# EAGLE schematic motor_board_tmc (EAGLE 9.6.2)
Assembly variants: ACS724, MAX503xD+ACS

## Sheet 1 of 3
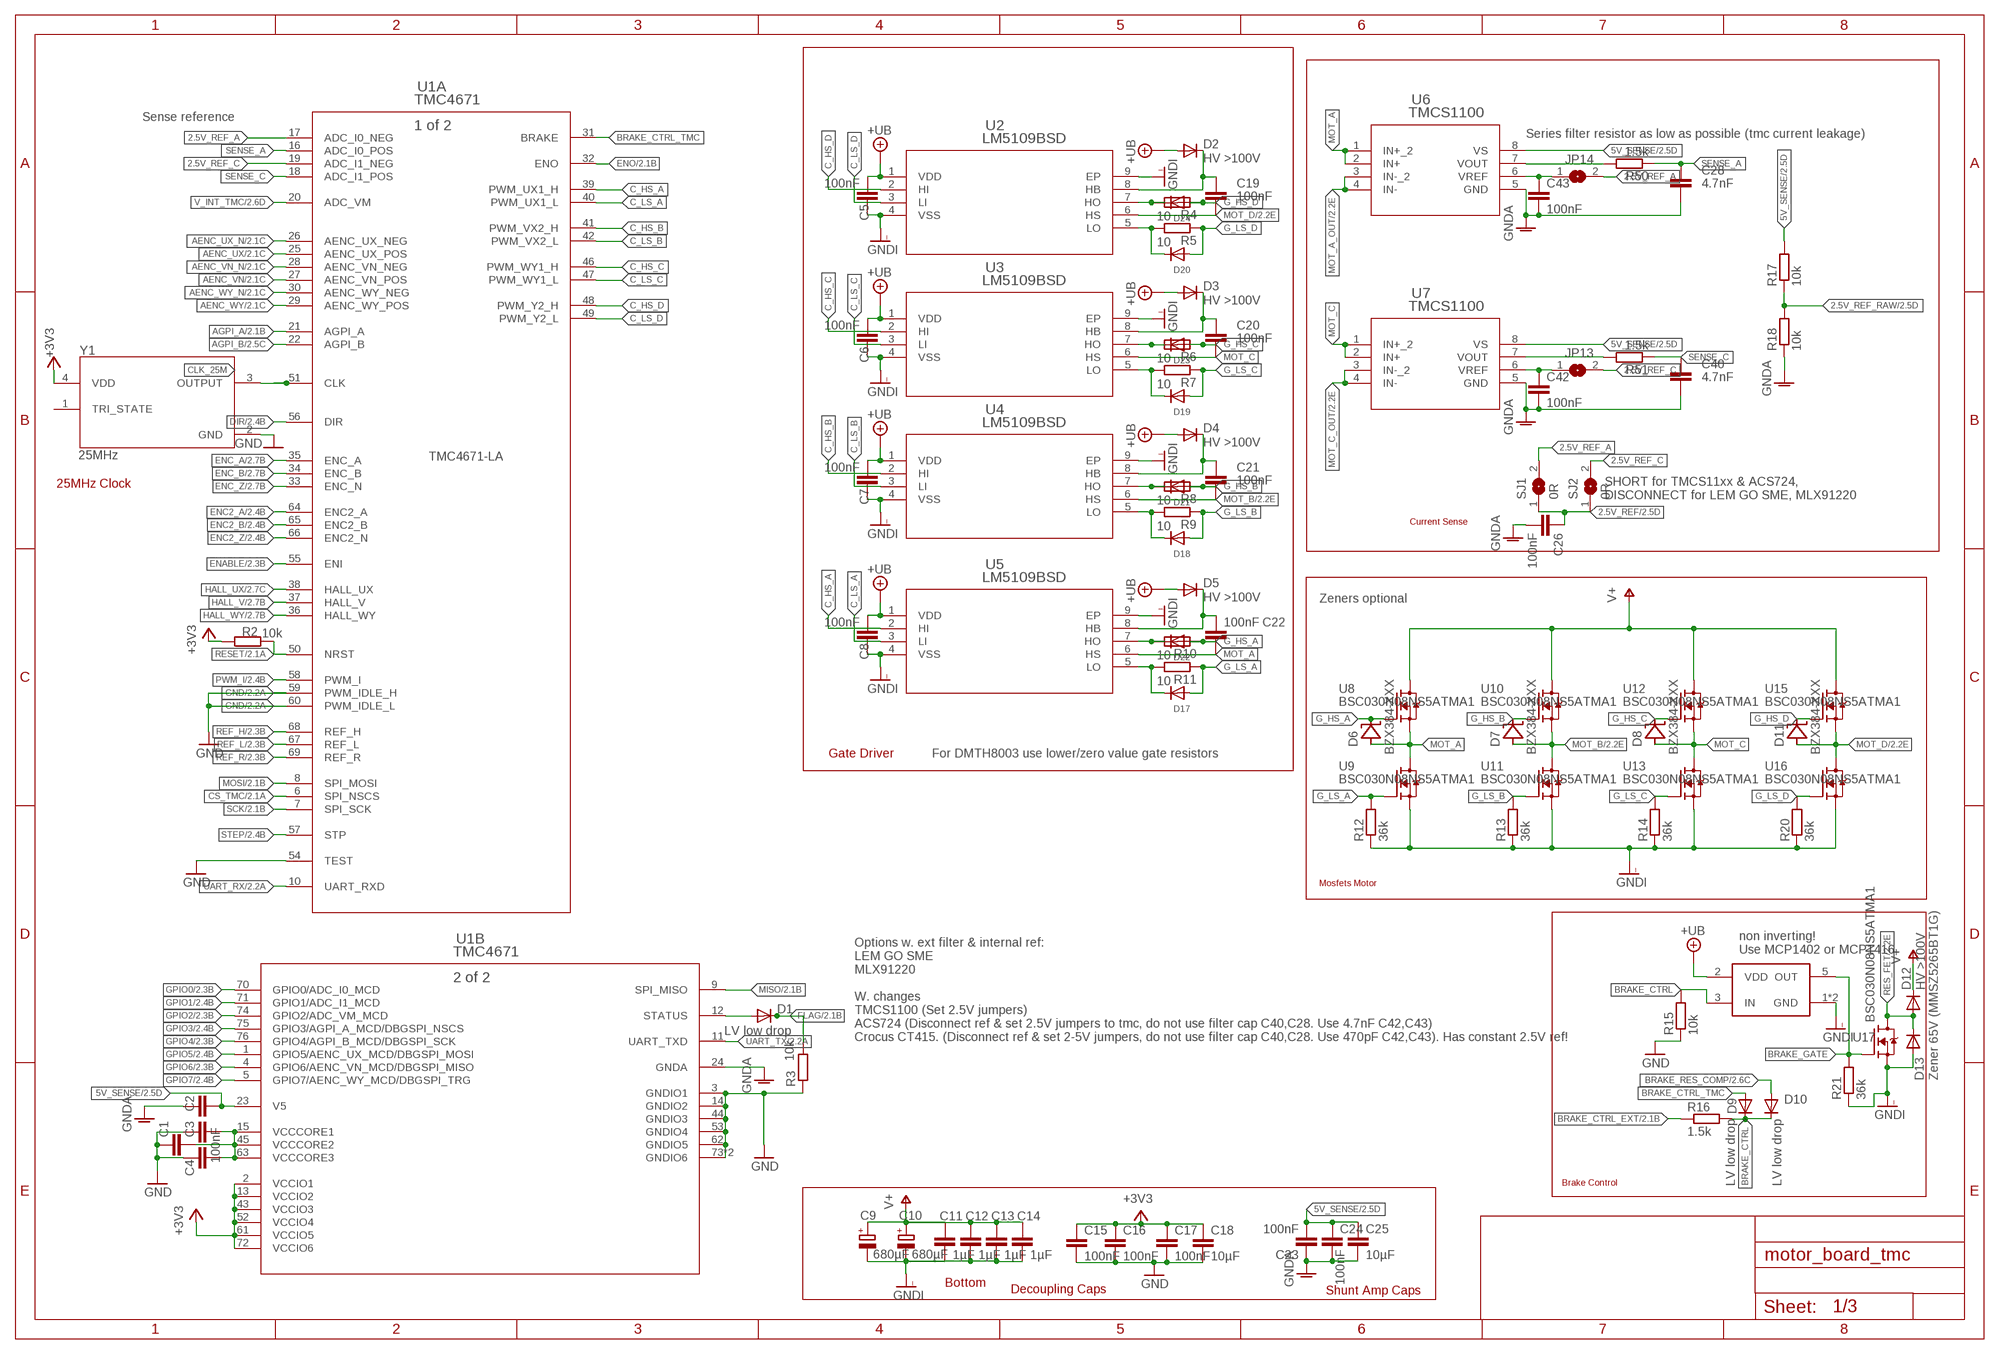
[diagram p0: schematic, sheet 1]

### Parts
C1  100nF  C-EUC0603  [C0603]
C2  10µF  C-EUC0805  [C0805]
C3  100nF  C-EUC0603  [C0603]
C4  100nF  C-EUC0603  [C0603]
C5  100nF  C-EUC0603  [C0603]
C6  100nF  C-EUC0603  [C0603]
C7  100nF  C-EUC0603  [C0603]
C8  100nF  C-EUC0603  [C0603]
C9  680µF  CPOL-EUE7.5-16  [E7,5-16]
C10  680µF  CPOL-EUE7.5-16  [E7,5-16]
C11  1µF  C-EUC1206  [C1206]
C12  1µF  C-EUC1206  [C1206]
C13  1µF  C-EUC1206  [C1206]
C14  1µF  C-EUC1206  [C1206]
C15  100nF  C-EUC0603  [C0603]
C16  100nF  C-EUC0603  [C0603]
C17  100nF  C-EUC0603  [C0603]
C18  10µF  C-EUC0805  [C0805]
C19  100nF  C-EUC0603  [C0603]
C20  100nF  C-EUC0603  [C0603]
C21  100nF  C-EUC0603  [C0603]
C22  100nF  C-EUC0603  [C0603]
C23  100nF  C-EUC0603  [C0603]
C24  100nF  C-EUC0603  [C0603]
C25  10µF  C-EUC0805  [C0805]
C26  100nF  C-EUC0603  [C0603]
C28  4.7nF  C-EUC0603  [C0603]  (not fitted in variant ACS724)  (not fitted in variant MAX503xD+ACS)
C40  4.7nF  C-EUC0603  [C0603]  (not fitted in variant ACS724)  (not fitted in variant MAX503xD+ACS)
C42  100nF  C-EUC0603  [C0603]  (variant ACS724: 4.7nF)  (variant MAX503xD+ACS: 4.7nF)
C43  100nF  C-EUC0603  [C0603]  (variant ACS724: 4.7nF)  (variant MAX503xD+ACS: 4.7nF)
D1  LV low drop  DIODE_SOD-123FL  [SOD-123FL]
D2  HV >100V  DIODE_SOD-123FL  [SOD-123FL]
D3  HV >100V  DIODE_SOD-123FL  [SOD-123FL]
D4  HV >100V  DIODE_SOD-123FL  [SOD-123FL]
D5  HV >100V  DIODE_SOD-123FL  [SOD-123FL]
D6  BZX384-XXX  [SOD323-R]
D7  BZX384-XXX  [SOD323-R]
D8  BZX384-XXX  [SOD323-R]
D9  LV low drop  DIODE_SOD-123FL  [SOD-123FL]
D10  LV low drop  DIODE_SOD-123FL  [SOD-123FL]
D11  BZX384-XXX  [SOD323-R]
D12  HV >100V  DIODE_SOD-123FL  [SOD-123FL]
D13  Zener 65V (MMSZ5265BT1G)  DIODE_SOD-123FL  [SOD-123FL]
D17  DIODESOD-323F  [SOD-323F]
D18  DIODESOD-323F  [SOD-323F]
D19  DIODESOD-323F  [SOD-323F]
D20  DIODESOD-323F  [SOD-323F]
D21  DIODESOD-323F  [SOD-323F]
D22  DIODESOD-323F  [SOD-323F]
D23  DIODESOD-323F  [SOD-323F]
D24  DIODESOD-323F  [SOD-323F]
JP13  JUMPER-SMT_2_NO_SILK  RESJUMPER0603  [RESISTOR_R0603]  (not fitted in variant ACS724)  (not fitted in variant MAX503xD+ACS)
JP14  JUMPER-SMT_2_NO_SILK  RESJUMPER0603  [RESISTOR_R0603]  (not fitted in variant ACS724)  (not fitted in variant MAX503xD+ACS)
R2  10k  R-EU_R0603  [R0603]
R3  10k  R-EU_R0603  [R0603]
R4  10  R-EU_R0603  [R0603]
R5  10  R-EU_R0603  [R0603]
R6  10  R-EU_R0603  [R0603]
R7  10  R-EU_R0603  [R0603]
R8  10  R-EU_R0603  [R0603]
R9  10  R-EU_R0603  [R0603]
R10  10  R-EU_R0603  [R0603]
R11  10  R-EU_R0603  [R0603]
R12  36k  R-EU_R0603  [R0603]
R13  36k  R-EU_R0603  [R0603]
R14  36k  R-EU_R0603  [R0603]
R15  10k  R-EU_R0603  [R0603]
R16  1.5k  R-EU_R0603  [R0603]
R17  10k  R-EU_R0603  [R0603]
R18  10k  R-EU_R0603  [R0603]
R20  36k  R-EU_R0603  [R0603]
R21  36k  R-EU_R0603  [R0603]
R50  1.5k  R-EU_R0603  [R0603]  (variant ACS724: 0)  (variant MAX503xD+ACS: 0)
R51  1.5k  R-EU_R0603  [R0603]  (variant ACS724: 0)  (variant MAX503xD+ACS: 0)
SJ1  0R  RESJUMPER0603  [RESISTOR_R0603]
SJ2  0R  RESJUMPER0603  [RESISTOR_R0603]
U1  TMC4671  [QFN76_10P5X6P5]
U2  LM5109BSD  [SDC08A]
U3  LM5109BSD  [SDC08A]
U4  LM5109BSD  [SDC08A]
U5  LM5109BSD  [SDC08A]
U6  TMCS1100  [SOIC8_D_TEX]
U7  TMCS1100  [SOIC8_D_TEX]
U8  BSC030N08NS5ATMA1  [MOSFET_BSC093N04LSGATMA1]
U9  BSC030N08NS5ATMA1  [MOSFET_BSC093N04LSGATMA1]
U10  BSC030N08NS5ATMA1  [MOSFET_BSC093N04LSGATMA1]
U11  BSC030N08NS5ATMA1  [MOSFET_BSC093N04LSGATMA1]
U12  BSC030N08NS5ATMA1  [MOSFET_BSC093N04LSGATMA1]
U13  BSC030N08NS5ATMA1  [MOSFET_BSC093N04LSGATMA1]
U14  MCP14XX  [SOT23-5L]
U15  BSC030N08NS5ATMA1  [MOSFET_BSC093N04LSGATMA1]
U16  BSC030N08NS5ATMA1  [MOSFET_BSC093N04LSGATMA1]
U17  BSC030N08NS5ATMA1  [MOSFET_BSC093N04LSGATMA1]
Y1  25MHz  ECS-327KE-TR  [ECS-327KE-TR]

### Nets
2.5V_REF: C26.1 SJ1.1 SJ2.1 ; also sheet 2
2.5V_REF_A: JP14.2 SJ1.2 U1.17(A:ADC_I0_NEG)
2.5V_REF_C: JP13.2 SJ2.2 U1.19(A:ADC_I1_NEG)
2.5V_REF_RAW: R17.1 R18.2 ; also sheet 2
5V_SENSE: C2.2 C23.2 C24.1 C25.1 R17.2 U1.23(B:V5) U6.8(VS) U7.8(VS) ; also sheet 2,3
+3V3: C15.1 C16.1 C17.1 C18.1 R2.2 U1.2(B:VCCIO1) U1.13(B:VCCIO2) U1.43(B:VCCIO3) U1.52(B:VCCIO4) U1.61(B:VCCIO5) U1.72(B:VCCIO6) Y1.4(VDD) ; also sheet 2,3
AENC_UX: U1.25(A:AENC_UX_POS) ; also sheet 2
AENC_UX_N: U1.26(A:AENC_UX_NEG) ; also sheet 2
AENC_VN: U1.27(A:AENC_VN_POS) ; also sheet 2
AENC_VN_N: U1.28(A:AENC_VN_NEG) ; also sheet 2
AENC_WY: U1.29(A:AENC_WY_POS) ; also sheet 2
AENC_WY_N: U1.30(A:AENC_WY_NEG) ; also sheet 2
AGPI_A: U1.21(A:AGPI_A) ; also sheet 2
AGPI_B: U1.22(A:AGPI_B) ; also sheet 2
BRAKE_CTRL: D9.C D10.C R15.2 R16.2 U14.3(IN)
BRAKE_CTRL_EXT: R16.1 ; also sheet 2
BRAKE_CTRL_TMC: D9.A U1.31(A:BRAKE)
BRAKE_GATE: R21.2 U14.5(OUT) U17.4(G)
BRAKE_RES_COMP: D10.A ; also sheet 2
C_HS_A: U1.39(A:PWM_UX1_H) U5.2(HI)
C_HS_B: U1.41(A:PWM_VX2_H) U4.2(HI)
C_HS_C: U1.46(A:PWM_WY1_H) U3.2(HI)
C_HS_D: U1.48(A:PWM_Y2_H) U2.2(HI)
C_LS_A: U1.40(A:PWM_UX1_L) U5.3(LI)
C_LS_B: U1.42(A:PWM_VX2_L) U4.3(LI)
C_LS_C: U1.47(A:PWM_WY1_L) U3.3(LI)
C_LS_D: U1.49(A:PWM_Y2_L) U2.3(LI)
CLK_25M: U1.51(A:CLK) Y1.3(OUTPUT)
CS_TMC: U1.6(A:SPI_NSCS) ; also sheet 2
DIR: U1.56(A:DIR) ; also sheet 2
ENABLE: U1.55(A:ENI) ; also sheet 2
ENC2_A: U1.64(A:ENC2_A) ; also sheet 2
ENC2_B: U1.65(A:ENC2_B) ; also sheet 2
ENC2_Z: U1.66(A:ENC2_N) ; also sheet 2
ENC_A: U1.35(A:ENC_A) ; also sheet 2
ENC_B: U1.34(A:ENC_B) ; also sheet 2
ENC_Z: U1.33(A:ENC_N) ; also sheet 2
ENO: U1.32(A:ENO) ; also sheet 2
FLAG: D1.C R3.2 ; also sheet 2
G_HS_A: D6.C D22.A R10.1 U8.4(G)
G_HS_B: D7.C D21.A R8.1 U10.4(G)
G_HS_C: D8.C D23.A R6.1 U12.4(G)
G_HS_D: D11.C D24.A R4.1 U15.4(G)
G_LS_A: D17.A R11.1 R12.2 U9.4(G)
G_LS_B: D18.A R9.1 R13.2 U11.4(G)
G_LS_C: D19.A R7.1 R14.2 U13.4(G)
G_LS_D: D20.A R5.1 R20.2 U16.4(G)
GND: C1.1 C3.1 C4.1 C15.2 C16.2 C17.2 C18.2 R3.1 R15.1 U1.3(B:GNDIO1) U1.14(B:GNDIO2) U1.44(B:GNDIO3) U1.53(B:GNDIO4) U1.54(A:TEST) U1.59(A:PWM_IDLE_H) U1.60(A:PWM_IDLE_L) U1.62(B:GNDIO5) U1.73(B:GNDIO6) U1.77(B:GNDIO6) Y1.2(GND) ; also sheet 2,3
GNDA: C2.1 C23.1 C24.2 C25.2 C26.2 C28.2 C40.2 C42.2 C43.2 R18.1 U1.24(B:GNDA) U6.5(GND) U7.5(GND) ; also sheet 2,3
GNDI [power]: C5.1 C6.1 C7.1 C8.1 C9.- C10.- C11.2 C12.2 C13.2 C14.2 D13.A R12.1 R13.1 R14.1 R20.1 R21.1 U2.4(VSS) U2.9(EP) U3.4(VSS) U3.9(EP) U4.4(VSS) U4.9(EP) U5.4(VSS) U5.9(EP) U9.1(S) U9.2(S) U9.3(S) U11.1(S) U11.2(S) U11.3(S) U13.1(S) U13.2(S) U13.3(S) U14.1(GND) U14.4(GND) U16.1(S) U16.2(S) U16.3(S) U17.1(S) U17.2(S) U17.3(S) ; also sheet 2,3
GPIO0: U1.70(B:GPIO0/ADC_I0_MCD) ; also sheet 2
GPIO1: U1.71(B:GPIO1/ADC_I1_MCD) ; also sheet 2
GPIO2: U1.74(B:GPIO2/ADC_VM_MCD) ; also sheet 2
GPIO3: U1.75(B:GPIO3/AGPI_A_MCD/DBGSPI_NSCS) ; also sheet 2
GPIO4: U1.76(B:GPIO4/AGPI_B_MCD/DBGSPI_SCK) ; also sheet 2
GPIO5: U1.1(B:GPIO5/AENC_UX_MCD/DBGSPI_MOSI) ; also sheet 2
GPIO6: U1.4(B:GPIO6/AENC_VN_MCD/DBGSPI_MISO) ; also sheet 2
GPIO7: U1.5(B:GPIO7/AENC_WY_MCD/DBGSPI_TRG) ; also sheet 2
HALL_UX: U1.38(A:HALL_UX) ; also sheet 2
HALL_V: U1.37(A:HALL_V) ; also sheet 2
HALL_WY: U1.36(A:HALL_WY) ; also sheet 2
MISO: U1.9(B:SPI_MISO) ; also sheet 2
MOSI: U1.8(A:SPI_MOSI) ; also sheet 2
MOT_A: C22.2 D6.A U5.6(HS) U6.1(IN+_2) U6.2(IN+) U8.1(S) U8.2(S) U8.3(S) U9.5(D)
MOT_A_OUT: U6.3(IN-_2) U6.4(IN-) ; also sheet 2
MOT_B: C21.2 D7.A U4.6(HS) U10.1(S) U10.2(S) U10.3(S) U11.5(D) ; also sheet 2
MOT_C: C20.2 D8.A U3.6(HS) U7.1(IN+_2) U7.2(IN+) U12.1(S) U12.2(S) U12.3(S) U13.5(D)
MOT_C_OUT: U7.3(IN-_2) U7.4(IN-) ; also sheet 2
MOT_D: C19.2 D11.A U2.6(HS) U15.1(S) U15.2(S) U15.3(S) U16.5(D) ; also sheet 2
N$4: D1.A U1.12(B:STATUS)
N$13: D17.C R11.2 U5.5(LO)
N$18: C22.1 D5.C U5.8(HB)
N$27: D22.C R10.2 U5.7(HO)
N$28: C21.1 D4.C U4.8(HB)
N$29: D18.C R9.2 U4.5(LO)
N$30: D21.C R8.2 U4.7(HO)
N$31: C19.1 D2.C U2.8(HB)
N$32: D20.C R5.2 U2.5(LO)
N$33: D24.C R4.2 U2.7(HO)
N$34: C20.1 D3.C U3.8(HB)
N$35: D19.C R7.2 U3.5(LO)
N$36: D23.C R6.2 U3.7(HO)
PWM_I: U1.58(A:PWM_I) ; also sheet 2
REF_H: U1.68(A:REF_H) ; also sheet 2
REF_L: U1.67(A:REF_L) ; also sheet 2
REF_R: U1.69(A:REF_R) ; also sheet 2
RES_FET: D12.A D13.C U17.5(D) ; also sheet 2
RESET: R2.1 U1.50(A:NRST) ; also sheet 2
SCK: U1.7(A:SPI_SCK) ; also sheet 2
SENSE_A: C28.1 R50.1 U1.16(A:ADC_I0_POS)
SENSE_A_RAW: R50.2 U6.7(VOUT)
SENSE_C: C40.1 R51.1 U1.18(A:ADC_I1_POS)
SENSE_C_RAW: R51.2 U7.7(VOUT)
STEP: U1.57(A:STP) ; also sheet 2
UART_RX: U1.10(A:UART_RXD) ; also sheet 2
UART_TX: U1.11(B:UART_TXD) ; also sheet 2
V+ [power]: C9.+ C10.+ C11.1 C12.1 C13.1 C14.1 D12.C U8.5(D) U10.5(D) U12.5(D) U15.5(D) ; also sheet 2,3
V_GD: C5.2 C6.2 C7.2 C8.2 D2.A D3.A D4.A D5.A U2.1(VDD) U3.1(VDD) U4.1(VDD) U5.1(VDD) U14.2(VDD) ; supply symbol labelled +UB ; also sheet 2,3
V_INT_TMC: U1.20(A:ADC_VM) ; also sheet 2
VCORE: C1.2 C3.2 C4.2 U1.15(B:VCCCORE1) U1.45(B:VCCCORE2) U1.63(B:VCCCORE3)
VREF_A_RAW: C43.1 JP14.1 U6.6(VREF)
VREF_C_RAW: C42.1 JP13.1 U7.6(VREF)
Unconnected: Y1.1(TRI_STATE)

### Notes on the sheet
- Sense reference
- Series filter resistor as low as possible (tmc current leakage)
- TMC4671-LA
- 25MHz Clock
- SHORT for TMCS11xx & ACS724,
  DISCONNECT for LEM GO SME, MLX91220
- Current Sense
- Zeners optional
- Gate Driver | For DMTH8003 use lower/zero value gate resistors
- Mosfets Motor
- non inverting!
  Use MCP1402 or MCP1416
- Options w. ext filter & internal ref:
  LEM GO SME
  MLX91220
  
  W. changes
  TMCS1100 (Set 2.5V jumpers)
  ACS724 (Disconnect ref & set 2.5V jumpers to tmc, do not use filter cap C40,C28. Use 4.7nF C42,C43)
  Crocus CT415. (Disconnect ref & set 2-5V jumpers, do not use filter cap C40,C28. Use 470pF C42,C43). Has constant 2.5V ref!
- Brake Control
- Bottom
- Decoupling Caps | Shunt Amp Caps

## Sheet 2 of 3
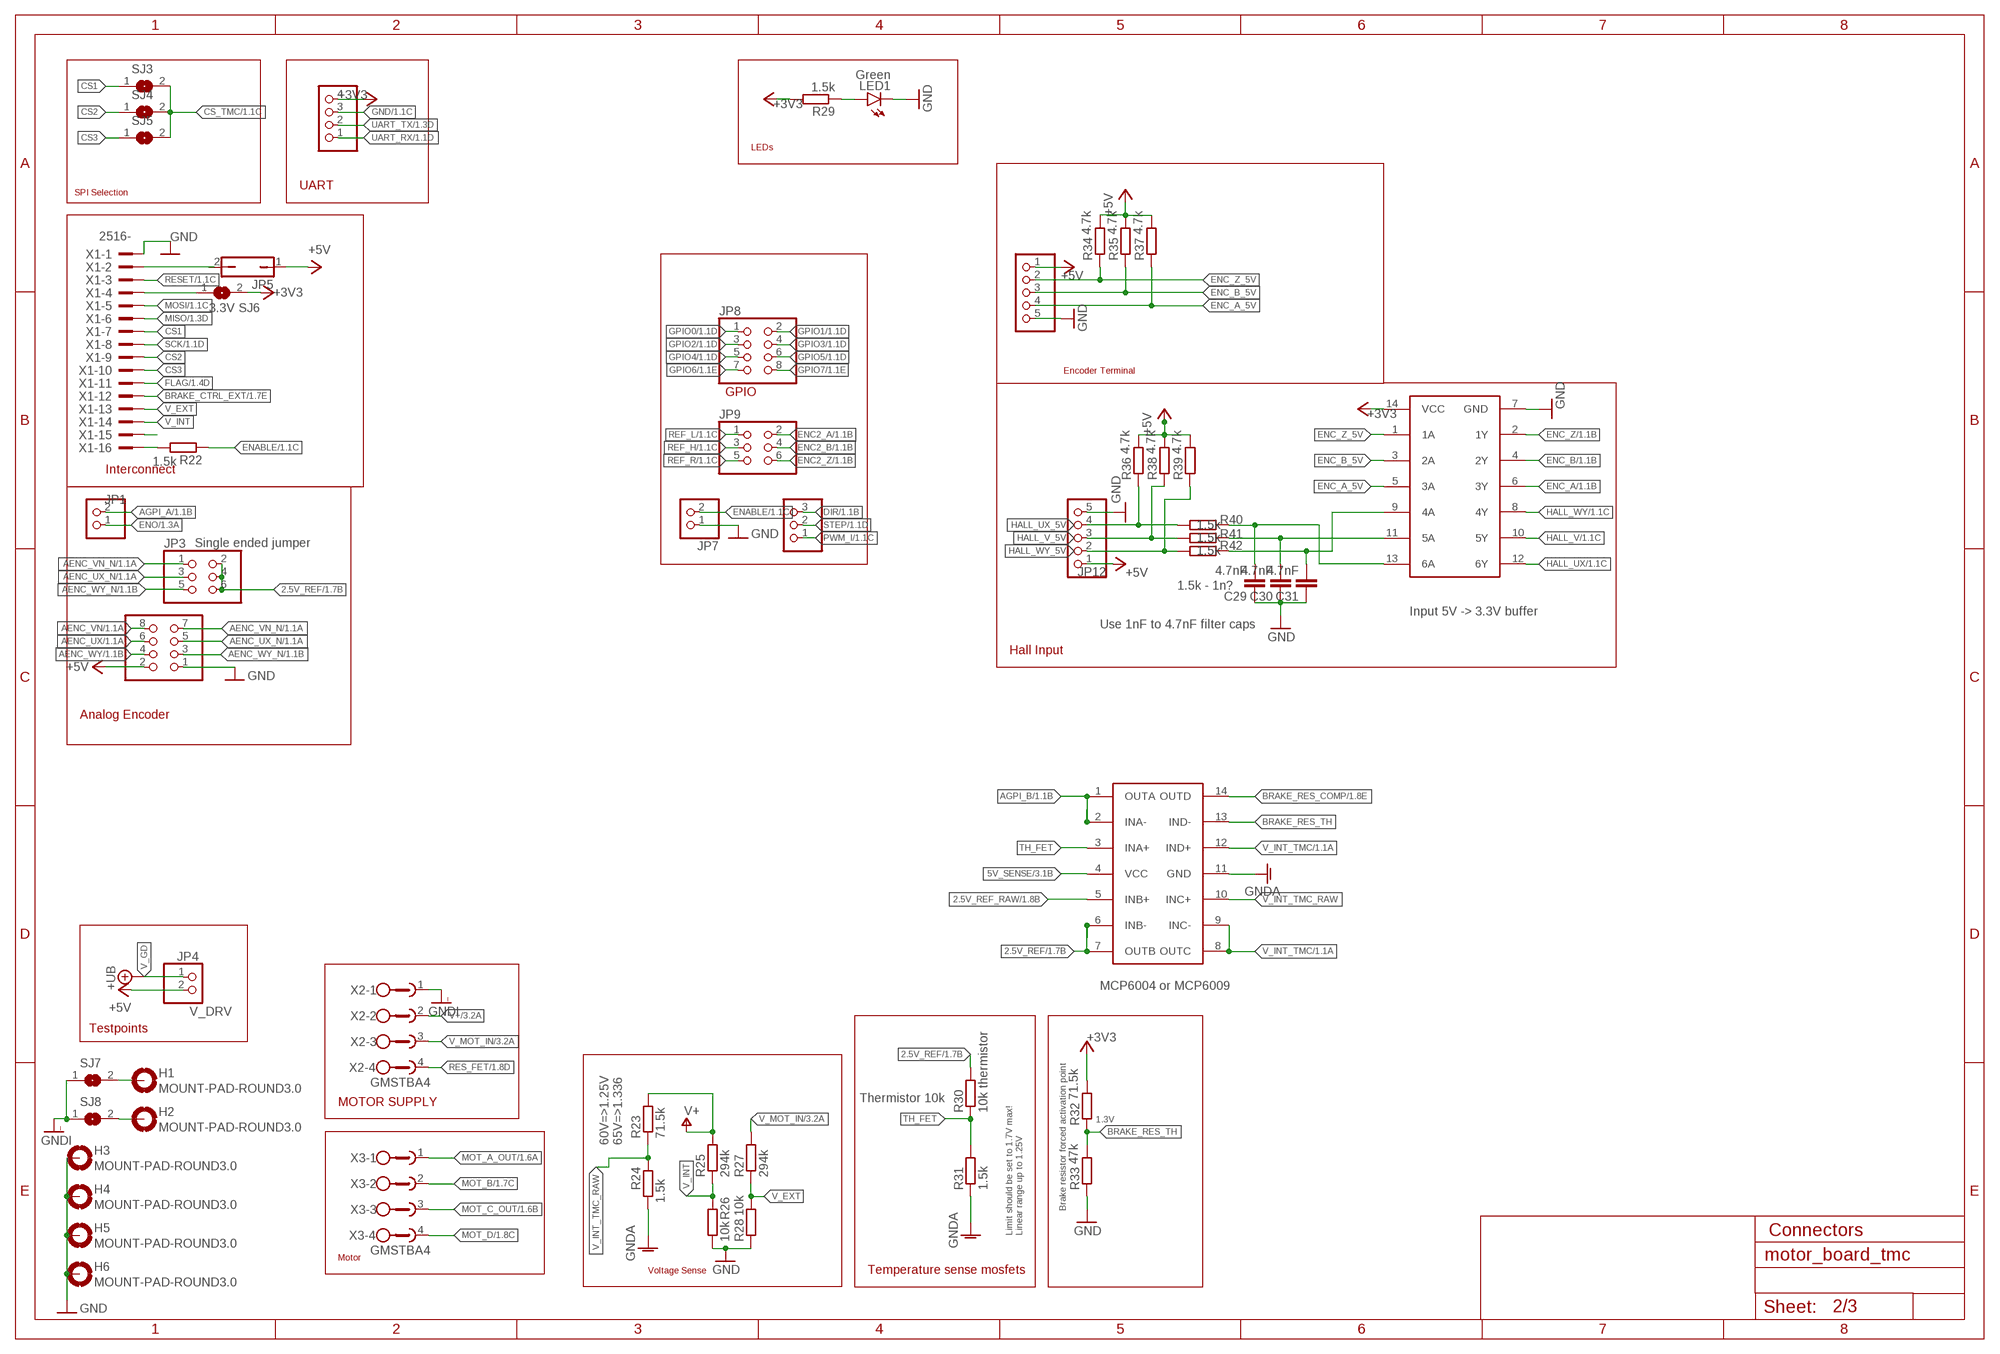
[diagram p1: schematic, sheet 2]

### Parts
C29  4.7nF  C-EUC0603  [C0603]
C30  4.7nF  C-EUC0603  [C0603]
C31  4.7nF  C-EUC0603  [C0603]
H1  MOUNT-PAD-ROUND3.0  [3,0-PAD]
H2  MOUNT-PAD-ROUND3.0  [3,0-PAD]
H3  MOUNT-PAD-ROUND3.0  [3,0-PAD]
H4  MOUNT-PAD-ROUND3.0  [3,0-PAD]
H5  MOUNT-PAD-ROUND3.0  [3,0-PAD]
H6  MOUNT-PAD-ROUND3.0  [3,0-PAD]
JP1  PINHD-1X2  [1X02]
JP2  PINHD-2X4  [2X04]
JP3  PINHD-2X3  [2X03]
JP4  V_DRV  PINHD-1X2  [1X02]
JP5  JP1Q  [JP1]
JP6  PINHD-1X4  [1X04]
JP7  PINHD-1X2  [1X02]
JP8  PINHD-2X4  [2X04]
JP9  PINHD-2X3  [2X03]
JP10  PINHD-1X3  [1X03]
JP11  PINHD-1X5  [1X05]
JP12  PINHD-1X5  [1X05]
LED1  Green  LEDSML0805  [SML0805]
R22  1.5k  R-EU_R0603  [R0603]
R23  71.5k  R-EU_R0805  [R0805]
R24  1.5k  R-EU_R0603  [R0603]
R25  294k  R-EU_R0805  [R0805]
R26  10k  R-EU_R0603  [R0603]
R27  294k  R-EU_R0805  [R0805]
R28  10k  R-EU_R0603  [R0603]
R29  1.5k  R-EU_R0603  [R0603]
R30  10k thermistor  R-EU_R0603  [R0603]
R31  1.5k  R-EU_R0603  [R0603]
R32  71.5k  R-EU_R0805  [R0805]
R33  47k  R-EU_R0603  [R0603]
R34  4.7k  R-EU_R0603  [R0603]
R35  4.7k  R-EU_R0603  [R0603]
R36  4.7k  R-EU_R0603  [R0603]
R37  4.7k  R-EU_R0603  [R0603]
R38  4.7k  R-EU_R0603  [R0603]
R39  4.7k  R-EU_R0603  [R0603]
R40  1.5k  R-EU_R0603  [R0603]
R41  1.5k  R-EU_R0603  [R0603]
R42  1.5k  R-EU_R0603  [R0603]
SJ3  SJ  [SJ]
SJ4  SJ  [SJ]
SJ5  SJ  [SJ]
SJ6  3.3V  SJ  [SJ]
SJ7  SJ  [SJ]
SJ8  SJ  [SJ]
U18  MCP6004  [TSSOP14]
U19  74LV17APWJ  [TSSOP14]
X1  2516-  [PAK100/2500-16]
X2  GMSTBA4  [GMSTBA4]
X3  GMSTBA4  [GMSTBA4]

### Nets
2.5V_REF: JP3.2 JP3.4 JP3.6 R30.2 U18.6(INB-) U18.7(OUTB) ; also sheet 1
2.5V_REF_RAW: U18.5(INB+) ; also sheet 1
5V_SENSE: U18.4(VCC) ; also sheet 1,3
+3V3: JP6.4 R29.2 R32.2 SJ6.2 U19.14(VCC) ; also sheet 1,3
+5V: JP2.2 JP4.2 JP5.1 JP11.1 JP12.1 R34.2 R35.2 R36.2 R37.2 R38.2 R39.2 ; also sheet 3
AENC_UX: JP2.6 ; also sheet 1
AENC_UX_N: JP2.5 JP3.3 ; also sheet 1
AENC_VN: JP2.8 ; also sheet 1
AENC_VN_N: JP2.7 JP3.1 ; also sheet 1
AENC_WY: JP2.4 ; also sheet 1
AENC_WY_N: JP2.3 JP3.5 ; also sheet 1
AGPI_A: JP1.2 ; also sheet 1
AGPI_B: U18.1(OUTA) U18.2(INA-) ; also sheet 1
BRAKE_CTRL_EXT: X1.12 ; also sheet 1
BRAKE_RES_COMP: U18.14(OUTD) ; also sheet 1
BRAKE_RES_TH: R32.1 R33.2 U18.13(IND-)
CS1: SJ3.1 X1.7
CS2: SJ4.1 X1.9
CS3: SJ5.1 X1.10
CS_TMC: SJ3.2 SJ4.2 SJ5.2 ; also sheet 1
DIR: JP10.3 ; also sheet 1
ENABLE: JP7.2 R22.1 ; also sheet 1
ENC2_A: JP9.2 ; also sheet 1
ENC2_B: JP9.4 ; also sheet 1
ENC2_Z: JP9.6 ; also sheet 1
ENC_A: U19.6(3Y) ; also sheet 1
ENC_A_5V: JP11.4 R37.1 U19.5(3A)
ENC_B: U19.4(2Y) ; also sheet 1
ENC_B_5V: JP11.3 R35.1 U19.3(2A)
ENC_Z: U19.2(1Y) ; also sheet 1
ENC_Z_5V: JP11.2 R34.1 U19.1(1A)
ENO: JP1.1 ; also sheet 1
FLAG: X1.11 ; also sheet 1
GND: C29.1 C30.1 C31.1 H3.B3,0(MOUNT) H4.B3,0(MOUNT) H5.B3,0(MOUNT) H6.B3,0(MOUNT) JP2.1 JP6.3 JP7.1 JP11.5 JP12.5 LED1.C R26.1 R28.1 R33.1 U19.7(GND) X1.1 ; also sheet 1,3
GNDA: R24.1 R31.1 U18.11(GND) ; also sheet 1,3
GNDI [power]: SJ7.1 SJ8.1 X2.1 ; also sheet 1,3
GPIO0: JP8.1 ; also sheet 1
GPIO1: JP8.2 ; also sheet 1
GPIO2: JP8.3 ; also sheet 1
GPIO3: JP8.4 ; also sheet 1
GPIO4: JP8.5 ; also sheet 1
GPIO5: JP8.6 ; also sheet 1
GPIO6: JP8.7 ; also sheet 1
GPIO7: JP8.8 ; also sheet 1
HALL_UX: U19.12(6Y) ; also sheet 1
HALL_UX_5V: C29.2 R40.1 U19.13(6A)
HALL_V: U19.10(5Y) ; also sheet 1
HALL_V_5V: C30.2 R41.1 U19.11(5A)
HALL_WY: U19.8(4Y) ; also sheet 1
HALL_WY_5V: C31.2 R42.1 U19.9(4A)
MISO: X1.6 ; also sheet 1
MOSI: X1.5 ; also sheet 1
MOT_A_OUT: X3.1 ; also sheet 1
MOT_B: X3.2 ; also sheet 1
MOT_C_OUT: X3.3 ; also sheet 1
MOT_D: X3.4 ; also sheet 1
N$1: JP12.4 R36.1 R40.2
N$2: X1.15
N$3: JP12.3 R38.1 R41.2
N$7: H1.B3,0(MOUNT) SJ7.2
N$8: LED1.A R29.1
N$9: JP5.2 X1.2
N$10: H2.B3,0(MOUNT) SJ8.2
N$15: JP12.2 R39.1 R42.2
N$17: R22.2 X1.16
N$20: SJ6.1 X1.4
PWM_I: JP10.1 ; also sheet 1
REF_H: JP9.3 ; also sheet 1
REF_L: JP9.1 ; also sheet 1
REF_R: JP9.5 ; also sheet 1
RES_FET: X2.4 ; also sheet 1
RESET: X1.3 ; also sheet 1
SCK: X1.8 ; also sheet 1
STEP: JP10.2 ; also sheet 1
TH_FET: R30.1 R31.2 U18.3(INA+)
UART_RX: JP6.1 ; also sheet 1
UART_TX: JP6.2 ; also sheet 1
V+ [power]: R23.2 R25.2 X2.2 ; also sheet 1,3
V_EXT: R27.1 R28.2 X1.13
V_GD: JP4.1 ; supply symbol labelled +UB ; also sheet 1,3
V_INT: R25.1 R26.2 X1.14
V_INT_TMC: U18.8(OUTC) U18.9(INC-) U18.12(IND+) ; also sheet 1
V_INT_TMC_RAW: R23.1 R24.2 U18.10(INC+)
V_MOT_IN: R27.2 X2.3 ; also sheet 3

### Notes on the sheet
- LEDs
- UART
- SPI Selection
- Encoder Terminal
- GPIO
- Interconnect
- Single ended jumper
- 1.5k - 1n?
- Input 5V -> 3.3V buffer
- Use 1nF to 4.7nF filter caps
- Hall Input
- Analog Encoder
- MCP6004 or MCP6009
- Testpoints
- Thermistor 10k
- MOTOR SUPPLY
- 1.3V
- 60V=>1.25V
  65V=>1.336
- Brake resistor forced activation point
- Limit should be set to 1.7V max!
  Linear range up to 1.25V
- Connectors
- Motor
- Voltage Sense | Temperature sense mosfets

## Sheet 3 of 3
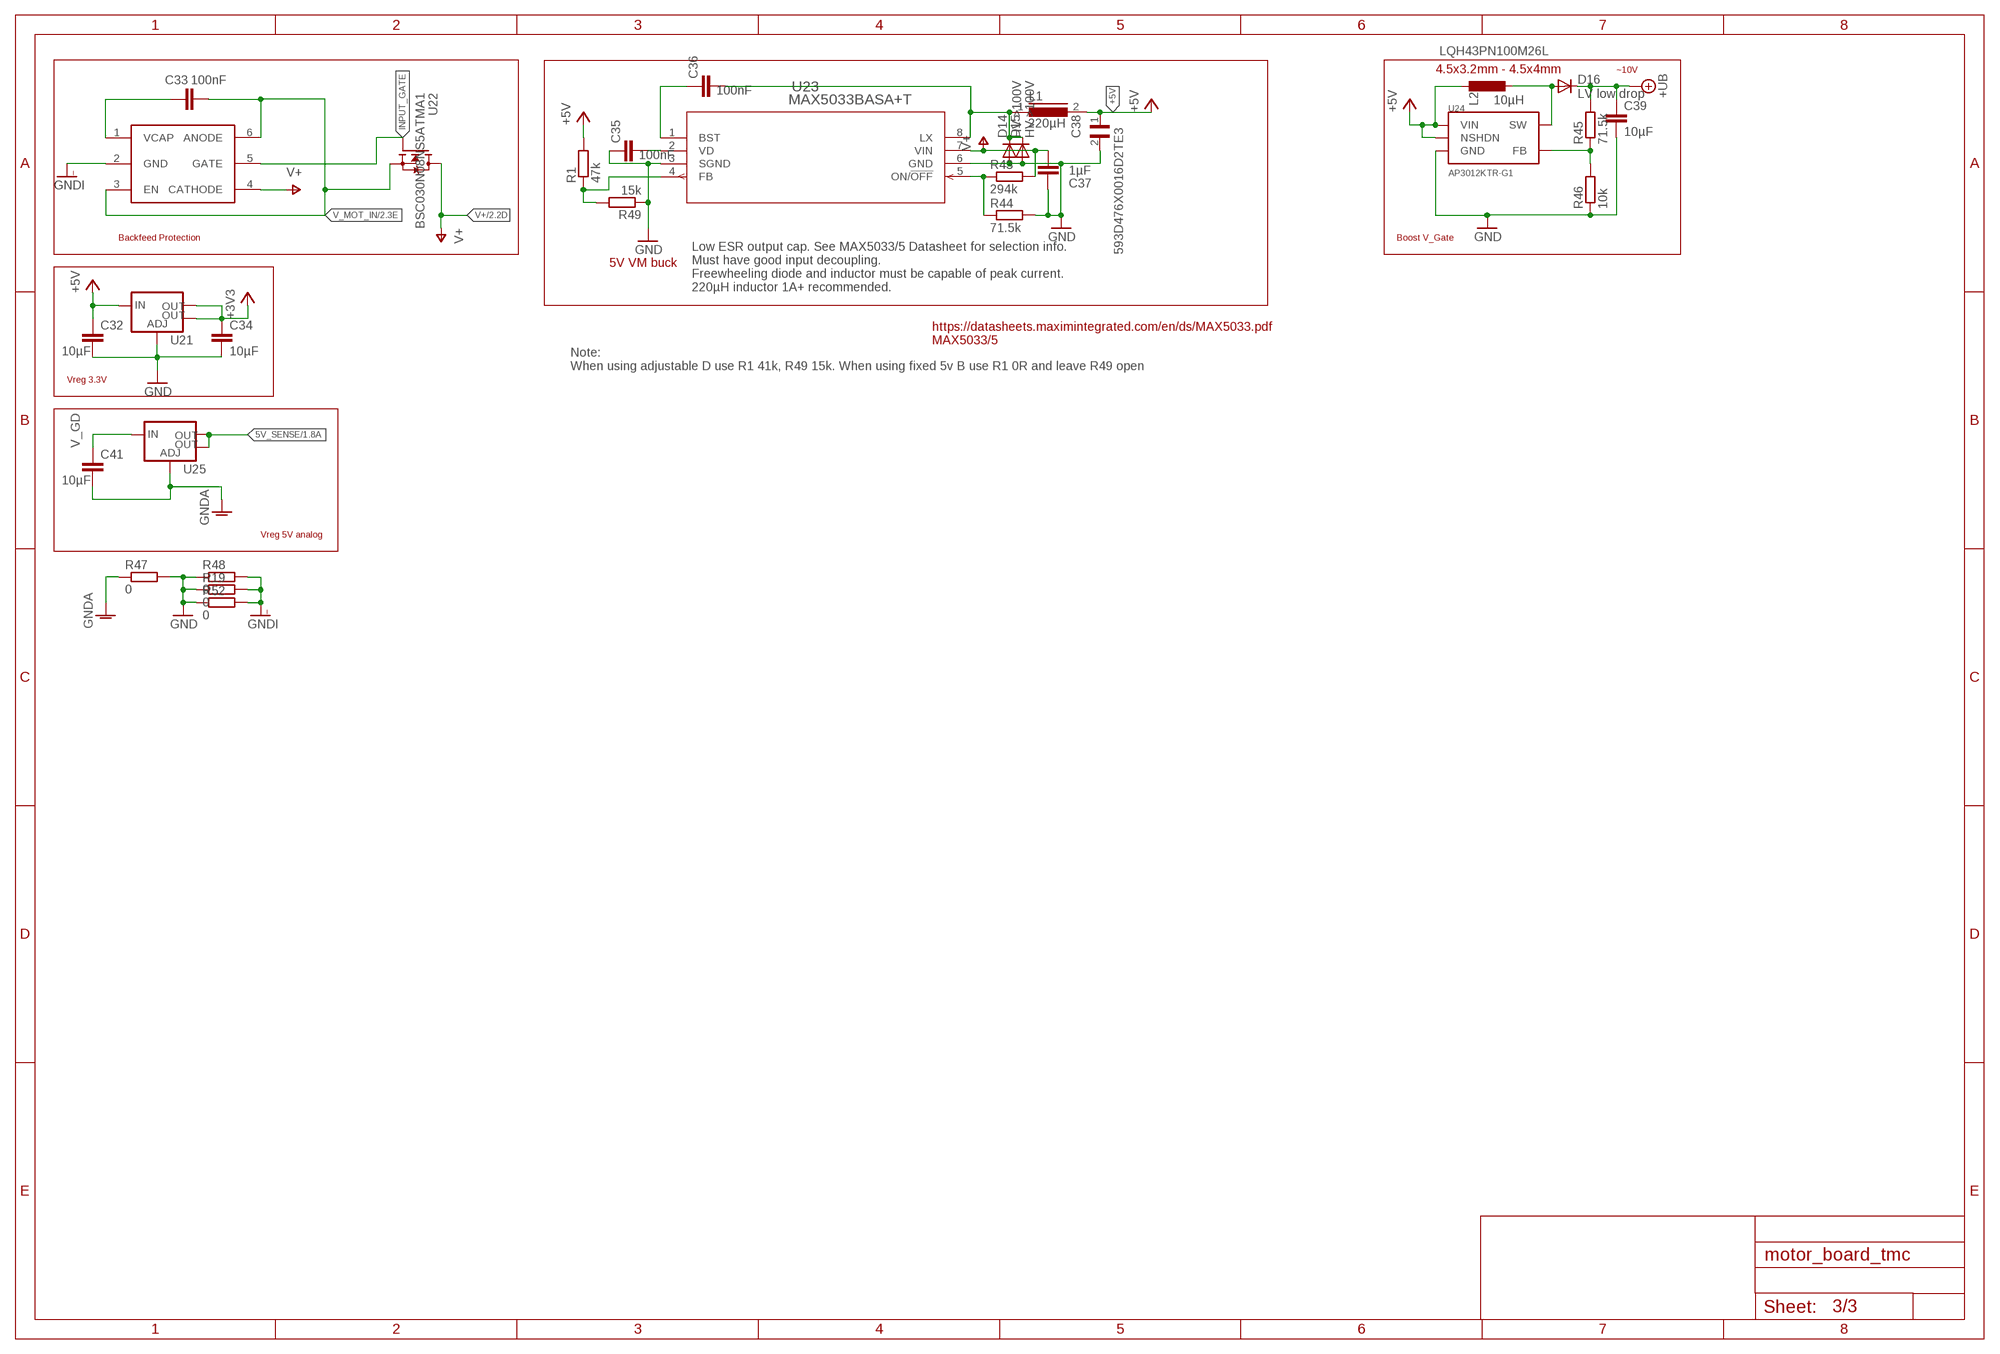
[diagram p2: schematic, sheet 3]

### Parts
C32  10µF  C-EUC0805  [C0805]
C33  100nF  C-EUC0603  [C0603]
C34  10µF  C-EUC0805  [C0805]
C35  100nF  C-EUC0603  [C0603]
C36  100nF  C-EUC0603  [C0603]
C37  1µF  C-EUC1206  [C1206]
C38  593D476X0016D2TE3  [CAPPM7343X310N]
C39  10µF  C-EUC0805  [C0805]
C41  10µF  C-EUC0805  [C0805]
D14  HV >100V  DIODE_SOD-123FL  [SOD-123FL]
D15  HV >100V  DIODESMA  [SMADIODE]
D16  LV low drop  DIODE_SOD-123FL  [SOD-123FL]
L1  220µH  8MMINDUCTOR  [8MMINDUCTOR]
L2  10µH  L-EUL4532P  [L4532P]
R1  47k  R-EU_R0603  [R0603]  (variant ACS724: 0)
R19  0  R-EU_R0603  [R0603]  (not fitted in variant ACS724)  (not fitted in variant MAX503xD+ACS)
R43  294k  R-EU_R0805  [R0805]
R44  71.5k  R-EU_R0805  [R0805]
R45  71.5k  R-EU_R0805  [R0805]
R46  10k  R-EU_R0603  [R0603]
R47  0  R-EU_R0603  [R0603]
R48  0  R-EU_R0603  [R0603]
R49  15k  R-EU_R0603  [R0603]  (not fitted in variant ACS724)
R52  0  R-EU_R0603  [R0603]  (not fitted in variant ACS724)  (not fitted in variant MAX503xD+ACS)
U20  LM74700-Q1  [SOT23-6]
U21  V_REG_LM1117SOT223  [SOT223]
U22  BSC030N08NS5ATMA1  [MOSFET_BSC093N04LSGATMA1]
U23  MAX5033BASA+T  [21-0041B_8_MXM]
U24  AP3012KTR-G1  [SOT23-5L]
U25  V_REG_LM1117SOT223  [SOT223]

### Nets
5V_SENSE: U25.2(OUT) U25.4(OUT) ; also sheet 1,2
+3V3: C34.1 U21.2(OUT) U21.4(OUT) ; also sheet 1,2
+5V: C32.1 C38.1 L1.2 L2.1 R1.2 U21.3(IN) U24.4(NSHDN) U24.5(VIN) ; also sheet 2
GND: C32.2 C34.2 C35.1 C37.1 C38.2 C39.2 D14.A D15.A R19.1 R44.2 R46.1 R47.2 R48.1 R49.1 R52.1 U21.1(ADJ) U23.3(SGND) U23.6(GND) U24.2(GND) ; also sheet 1,2
GNDA: C41.2 R47.1 U25.1(ADJ) ; also sheet 1,2
GNDI [power]: R19.2 R48.2 R52.2 U20.2(GND) ; also sheet 1,2
INPUT_GATE: U20.5(GATE) U22.4(G)
N$5: R45.1 R46.2 U24.3(FB)
N$6: R1.1 R49.2 U23.4(FB)
N$12: D16.A L2.2 U24.1(SW)
N$16: C36.2 D14.C D15.C L1.1 U23.8(LX)
N$19: C36.1 U23.1(BST)
N$21: R43.1 R44.1 U23.5(ON/!OFF)
N$24: C33.1 U20.1(VCAP)
N$25: C35.2 U23.2(VD)
V+ [power]: C37.2 R43.2 U20.4(CATHODE) U22.5(D) U23.7(VIN) ; also sheet 1,2
V_GD: C39.1 C41.1 D16.C R45.2 U25.3(IN) ; supply symbol labelled +UB ; also sheet 1,2
V_MOT_IN: C33.2 U20.3(EN) U20.6(ANODE) U22.1(S) U22.2(S) U22.3(S) ; also sheet 2

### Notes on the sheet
- LQH43PN100M26L
- 4.5x3.2mm - 4.5x4mm | ~10V
- Backfeed Protection | Boost V_Gate
- 5V VM buck
- Low ESR output cap. See MAX5033/5 Datasheet for selection info.
  Must have good input decoupling.
  Freewheeling diode and inductor must be capable of peak current.
  220µH inductor 1A+ recommended.
- https://datasheets.maximintegrated.com/en/ds/MAX5033.pdf
  MAX5033/5
- Note:
  When using adjustable D use R1 41k, R49 15k. When using fixed 5v B use R1 0R and leave R49 open
- Vreg 3.3V
- Vreg 5V analog

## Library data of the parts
C1-C8 C11-C26 C28-C37 C39-C43 = resistor:C-EU: CAPACITOR, European symbol
C9 C10 = resistor:CPOL-EU: POLARIZED CAPACITOR, European symbol
C38 = Powermisc:593D476X0016D2TE3: 593D Series 47 uF ±20% 16 V Surface Mount Molded Solid Tantalum Capacitor; ARROW_ELECTRONICS-PURCHASE-URL: https://snapeda.com/shop?store=Arrow+Electronics&id=1736527; DESCRIPTION: 47µF Molded Tantalum Capacitors 16V 2917 (7343 Metric) 150mOhm; DIGI-KEY_PART_NUMBER: 718-2142-1-ND; MF: Vishay Sprague; MOUSER-PURCHASE-URL: https://snapeda.com/shop?store=Mouser&id=1736527; MP: 593D476X0016D2TE3; PACKAGE: 2917 Vishay
D1-D5 D9 D10 D12-D24 = adafruit:DIODE: Diode
D6-D8 D11 = Powermisc:BZX384-XXX
H1-H6 = holes:MOUNT-PAD-ROUND: MOUNTING PAD, round
JP1 JP4 JP7 = pinhead:PINHD-1X2: PIN HEADER
JP2 JP8 = pinhead:PINHD-2X4: PIN HEADER
JP3 JP9 = pinhead:PINHD-2X3: PIN HEADER
JP5 = jumper:JP1Q: JUMPER
JP6 = pinhead:PINHD-1X4: PIN HEADER
JP10 = pinhead:PINHD-1X3: PIN HEADER
JP11 JP12 = pinhead:PINHD-1X5: PIN HEADER
JP13 JP14 SJ1 SJ2 = motor_board_tmc:RESJUMPER
L1 = Powermisc:8MMINDUCTOR: Inductor; SPICEPREFIX: L
L2 = rcl:L-EU: INDUCTOR, European symbol; SPICEPREFIX: L
LED1 = led:LED: LED
R1-R52 = resistor:R-EU_: RESISTOR, European symbol
SJ3-SJ8 = jumper:SJ: SMD solder JUMPER
U1 = Trinamic:TMC4671; MANUFACTURER_PART_NUMBER: TMC4671ES; VENDOR: TRINAMIC
U2-U5 = Powermisc:LM5109BSD; MANUFACTURER_PART_NUMBER: lm5109bsd; VENDOR: Texas Instruments
U6 U7 = Powermisc:TMCS1100; BUILT_BY: EMA_Cory; COPYRIGHT: Copyright (C) 2018 Accelerated Designs. All rights reserved; DATASHEET: https://www.ti.com/lit/ds/symlink/tmcs1100.pdf?ts=1593546414862&ref_url=https%253A%252F%252Fwww.ti.com%252Fproduct%252FTMCS1100; MANUFACTURER_PART_NUMBER: TMCS1100AxQDR; SOURCELIBRARY: TI_2020-06-30; VENDOR: Texas Instruments
U8-U13 U15-U17 U22 = OHSC_Power:BSC030N08NS5ATMA1: None; AVAILABILITY: Unavailable; DESCRIPTION: N-Channel 80 V 100 A 3 mO 61 nC SMT OptiMOS Power Mosfet - SuperSO-8; MF: Infineon Technologies; MP: BSC030N08NS5ATMA1; PACKAGE: PowerTDFN-8 Infineon; PRICE: None
U14 = Powermisc:MCP14XX
U18 = Powermisc:MCP6004
U19 = Powermisc:74LV17APWJ
U20 = OHSC_Power:LM74700-Q1
U21 U25 = SparkFun-IC-Power:V_REG_LM1117: Voltage Regulator LM1117 Standard adjustable voltage regulator but in SMD form. Spark Fun Electronics SKU : COM-00595; PROD_ID: VREG-08170
U23 = Powermisc:MAX5033BASA+T; BUILT_BY: EMA_UL_Team; MANUFACTURER_PART_NUMBER: max5033basa+T; SOURCELIBRARY: Maxim_2014-06-20; VENDOR: Maxim Integrated Products
U24 = Powermisc:AP3012KTR-G1
X1 = con-3m:2516-: 3M (TM) Pak 100 4-Wall Header Source: 3M; OC_FARNELL: unknown; OC_NEWARK: unknown
X2 X3 = con-phoenix-762:GMSTBA4: PHOENIX; MF: FARNELL; MPN: 1757268; OC_FARNELL: 3705195; OC_NEWARK: 71C4163
Y1 = Crystals:ECS-327KE-TR: XTAL OSC XO 32.7680KHZ CMOS SMD Manufacturer's datasheet; CREATED_BY: PCBLayout.com; DIGIKEY_PART_NUMBER: XC1751TR-ND; MANUFACTURER: ECS Inc.; MPN: ECS-327KE-TR; PACKAGE: 4-SMD

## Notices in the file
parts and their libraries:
SparkFun-IC-Power: Licensing: Creative Commons ShareAlike 4.0 International - https://creativecommons.org/licenses/by-sa/4.0
